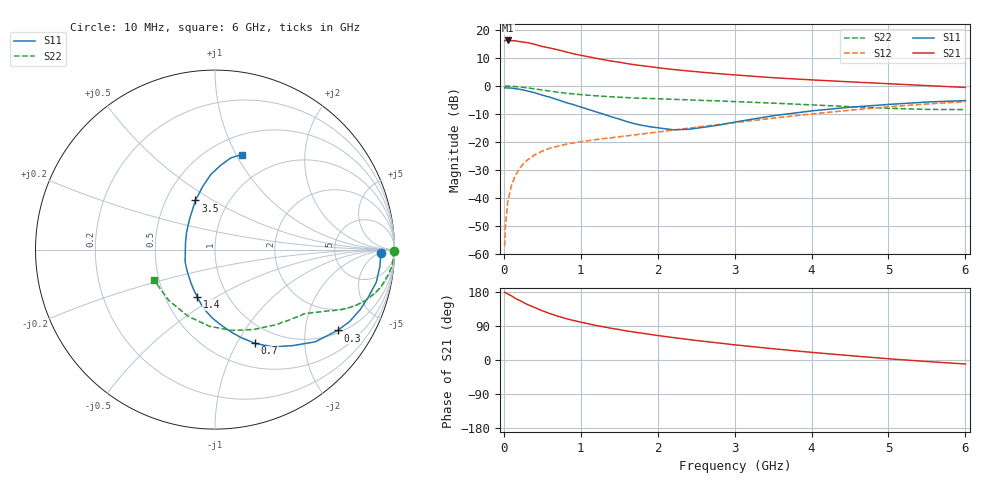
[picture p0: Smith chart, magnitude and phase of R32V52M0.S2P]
! SIEMENS Small Signal Semiconductors
! BFR181
! Si NPN RF Bipolar Junction Transistor in SOT23
! VCE = 2.5 V  IC = 2 mA
! Common Emitter S-Parameters:  May  1996
# GHz  S  MA  R  50
!  f  S11  S21  S12  S22
! GHz  MAG  ANG  MAG  ANG  MAG  ANG  MAG  ANG
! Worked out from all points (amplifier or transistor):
!   36 points, 10 MHz to 6 GHz, reference 50 ohm
!   highest |S21| = 16.2 dB at 50 MHz (marker M1)
!   |S21| within 3 dB of that: start of sweep to 648.8 MHz
!   unconditionally stable (mu >= 1): 1.579 GHz to 3.382 GHz
!   at 250 MHz: K = 0.23, MSG = 21.7 dB, |S12| = -27.8 dB
!   at 1.4 GHz: K = 0.95, MSG = 13.7 dB, |S12| = -18.4 dB
!   at 6 GHz: K = 0.86, MSG = 2.5 dB, |S12| = -5.6 dB
!   lowest NFmin = 1.35 dB at 450 MHz
!   S11 on the Smith chart (normalised r, x): 10 MHz: 24, -7; 300 MHz: 1.09, -2.97; 700 MHz: 0.77, -1.19; 1.4 GHz: 0.72, -0.41; 3.5 GHz: 0.70, +0.42; 6 GHz: 0.69, +1.05
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0.01  0.9265 -1.2  6.41 179.1  0.0014 94.6  0.9961 -0.6
0.02  0.9236 -2.4  6.465 177.5  0.0031 87.5  0.99 -1.1
0.05  0.9236 -5.7  6.471 174.4  0.0085 84.0  0.9942 -2.7
0.1  0.9168 -11.5  6.38 169.1  0.0171 83.5  0.9902 -5.3
0.15  0.8951 -17.0  6.381 162.6  0.0254 79.1  0.9759 -8.1
0.3  0.8183 -33.4  5.939 147.0  0.0473 71.0  0.9272 -14.8
0.4  0.7581 -42.7  5.528 138.6  0.0591 65.9  0.8875 -18.5
0.5  0.6868 -51.2  5.051 129.8  0.0693 62.3  0.8481 -21.3
0.6  0.6302 -59.3  4.744 122.5  0.0781 59.5  0.8113 -23.6
0.7  0.5685 -66.8  4.416 115.8  0.0845 57.1  0.7757 -25.6
0.8  0.5107 -73.6  4.081 109.7  0.0911 55.4  0.7466 -27.0
0.9  0.4668 -79.1  3.764 104.5  0.0966 54.3  0.722 -28.2
1.1  0.382 -92.2  3.317 95.5  0.1063 53.0  0.6844 -30.4
1.2  0.3451 -98.6  3.113 91.0  0.1109 52.8  0.6677 -31.5
1.4  0.2813 -110.5  2.772 83.5  0.1196 52.9  0.6419 -33.3
1.7  0.2125 -132.5  2.392 73.5  0.1344 54.3  0.6102 -35.9
2.2  0.1658 -176.0  1.967 59.2  0.1636 55.5  0.5782 -41.6
3  0.2271 127.7  1.575 40.0  0.2225 55.2  0.5268 -53.6
3.5  0.2948 111.7  1.404 29.7  0.2669 53.1  0.4946 -64.2
4.5  0.4183 93.3  1.184 11.5  0.3706 44.9  0.4286 -94.1
5.5  0.5177 80.3  1.015 -4.0  0.478 32.3  0.3825 -132.5
6  0.5498 74.4  0.943 -10.6  0.5259 25.0  0.3798 -153.4
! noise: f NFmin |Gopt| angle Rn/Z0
0.45  1.35  0.6  17  0.4
0.9  1.45  0.5  36  0.4
1.8  1.8  0.31  80  0.37
